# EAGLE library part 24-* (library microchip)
Serial EEPROM 32 K/64 K, 1.8 V, I2C
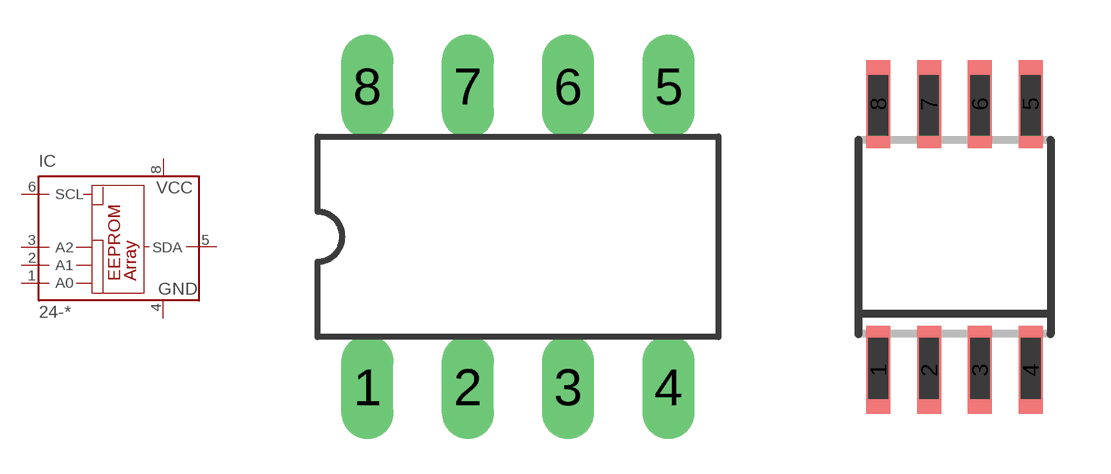
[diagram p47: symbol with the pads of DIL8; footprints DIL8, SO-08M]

Designator prefix IC

## 24-AA65P (MPN: 24AA65/P; OC_FARNELL: 1331306; OC_NEWARK: 35M0721), 24-C32P (MPN: AT24C32C-PU; OC_FARNELL: 1362652; OC_NEWARK: 50M3325), 24-C65P (MF: MICROCHIP; MPN: 24C65/P; OC_FARNELL: 9757821; OC_NEWARK: 89C9798), 24-FC32P (OC_FARNELL: unknown; OC_NEWARK: unknown), 24-FC65P (OC_FARNELL: unknown; OC_NEWARK: unknown), 24-LC32P (MF: MICROCHIP; MPN: 24LC32A/P; OC_FARNELL: 1084246; OC_NEWARK: 75K1884), 24-LC65P (MF: MICROCHIP; MPN: 24LC65/P; OC_FARNELL: 9758089; OC_NEWARK: 88K1357)  [DIL8]
1  A0  in
2  A1  in
3  A2  in
4  GND  pwr
5  SDA
6  SCL  in
8  VCC  pwr

## 24-AA65SM (MF: MICROCHIP; MPN: 24AA65/SM; OC_FARNELL: 1331307; OC_NEWARK: 92C6926), 24-C32SM (MPN: M24C32-WMN6P; OC_FARNELL: 1362654; OC_NEWARK: 56P9110), 24-C65SM (MF: MICROCHIP; MPN: 24C65/SM; OC_FARNELL: 1467721; OC_NEWARK: 96K4066), 24-FC32SM (OC_FARNELL: unknown; OC_NEWARK: unknown), 24-FC65SM (OC_FARNELL: unknown; OC_NEWARK: unknown), 24-LC32SM (MF: MICROCHIP; MPN: 24LC32A/SM; OC_FARNELL: 1212670; OC_NEWARK: 96K4080), 24-LC65SM (MF: MICROCHIP; MPN: 24LC65/SM; OC_FARNELL: 9758097; OC_NEWARK: 96K4082)  [SO-08M]
Pads as for DIL8

## Footprint DIL8 (pad centres in mm)
Dual In Line package type P
drill 0.813 long: 1 -3.81,-3.81; 2 -1.27,-3.81; 3 1.27,-3.81; 4 3.81,-3.81; 5 3.81,3.81; 6 1.27,3.81; 7 -1.27,3.81; 8 -3.81,3.81

## Footprint SO-08M (pad centres in mm)
Small Outline Medium Plastic Gull Wing 207-mil body, package type SM
smd 0.6 x 2.2: 1 -1.905,-3.33; 2 -0.635,-3.33; 3 0.635,-3.33; 4 1.905,-3.33; 5 1.905,3.33; 6 0.635,3.33; 7 -0.635,3.33; 8 -1.905,3.33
